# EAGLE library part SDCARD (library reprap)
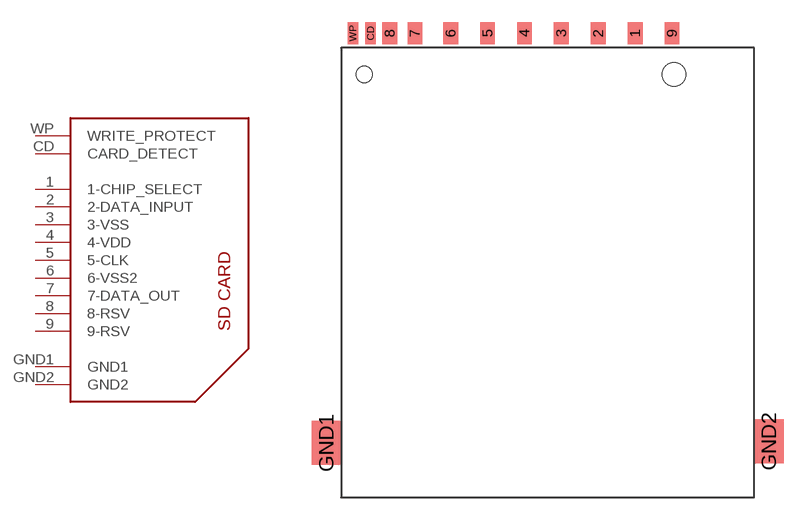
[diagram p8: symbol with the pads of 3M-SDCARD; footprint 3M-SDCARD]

Designator prefix -

## SDCARD  [3M-SDCARD]
1  1-CHIP_SELECT
2  2-DATA_INPUT
3  3-VSS
4  4-VDD
5  5-CLK
6  6-VSS2
7  7-DATA_OUT
8  8-RSV
9  9-RSV
CD  CARD_DETECT
GND1  GND1
GND2  GND2
WP  WRITE_PROTECT

## Footprint 3M-SDCARD (pad centres in mm)
smd 1 x 1.5: 1 5.93,16.5; 2 3.43,16.5; 3 0.93,16.5; 4 -1.57,16.5; 5 -4.07,16.5; 6 -6.57,16.5; 7 -9,16.5; 8 -10.7,16.5; 9 8.43,16.5
smd 0.7 x 1.5: CD -12,16.5; WP -13.2,16.5
smd 2 x 3: GND1 -15,-11.3; GND2 15,-11.2
hole 1.1 at -12.427,13.705
hole 1.6 at 8.567,13.708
